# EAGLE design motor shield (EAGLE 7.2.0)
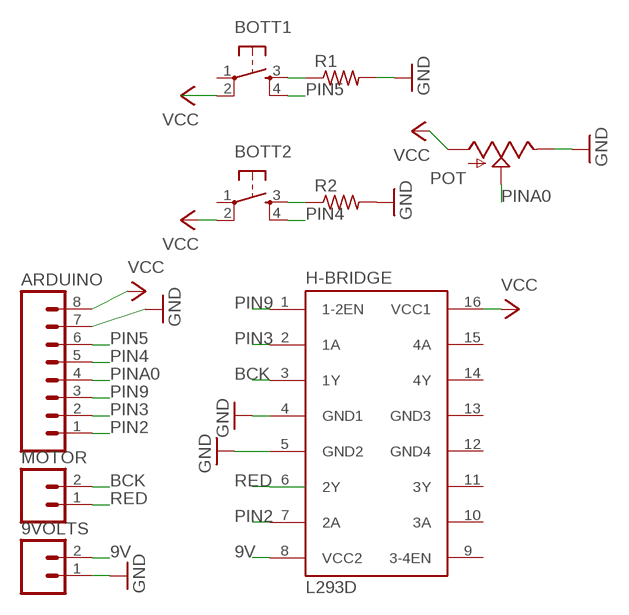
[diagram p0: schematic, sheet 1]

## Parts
9VOLTS  M02LOCK_LONGPADS  [1X02_LOCK_LONGPADS]
ARDUINO  M08LONGPADS  [1X08_LONGPADS]
BOTT1  6MM_SWITCH6MM_SWITCH  [6MM_SWITCH]
BOTT2  6MM_SWITCH6MM_SWITCH  [6MM_SWITCH]
H-BRIDGE  L293D  [DIL16]
MOTOR  M02LOCK_LONGPADS  [1X02_LOCK_LONGPADS]
POT  POT  [ALPS_POT]
R1  RESISTOR1206  [1206]
R2  RESISTOR1206  [1206]

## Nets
9V: 9VOLTS.2 H-BRIDGE.8(VCC2)
BCK: H-BRIDGE.3(1Y) MOTOR.2
GND: 9VOLTS.1 ARDUINO.7 H-BRIDGE.4(GND1) H-BRIDGE.5(GND2) POT.P$1(E) R1.2 R2.2
N$1: BOTT1.3(S) R1.1
N$2: BOTT2.3(S) R2.1
PIN2: ARDUINO.1 H-BRIDGE.7(2A)
PIN3: ARDUINO.2 H-BRIDGE.2(1A)
PIN4: ARDUINO.5 BOTT2.4(S1)
PIN5: ARDUINO.6 BOTT1.4(S1)
PIN9: ARDUINO.3 H-BRIDGE.1(1-2EN)
PINA0: ARDUINO.4 POT.P$2(S)
RED: H-BRIDGE.6(2Y) MOTOR.1
VCC: ARDUINO.8 BOTT1.2(P1) BOTT2.2(P1) H-BRIDGE.16(VCC1) POT.P$3(A)
Unconnected: BOTT1.1(P) BOTT2.1(P) H-BRIDGE.9(3-4EN) H-BRIDGE.10(3A) H-BRIDGE.11(3Y) H-BRIDGE.14(4Y) H-BRIDGE.15(4A)

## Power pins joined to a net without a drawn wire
GND3: H-BRIDGE.13(GND3)
GND4: H-BRIDGE.12(GND4)

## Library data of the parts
9VOLTS MOTOR = 01_SparkFun:M02: Header 2
ARDUINO = 01_SparkFun:M08: Header 8 Standard 8-pin 0.1" header. Use with straight break away headers (SKU : PRT-00116), right angle break away headers (PRT-00553), swiss pins (PRT-00743), machine pins (PRT-00117), and female headers (PRT-00115).
BOTT1 BOTT2 = 01_FAB_Hello:6MM_SWITCH: OMRON SWITCH
H-BRIDGE = st-microelectronics:L293D: PUSH-PULL 4 CHANNEL DRIVER; MPN: L293D; OC_FARNELL: 9589619; OC_NEWARK: 56P8249
POT = 01_SparkFun:POT
R1 R2 = 01_FAB_Hello:RESISTOR

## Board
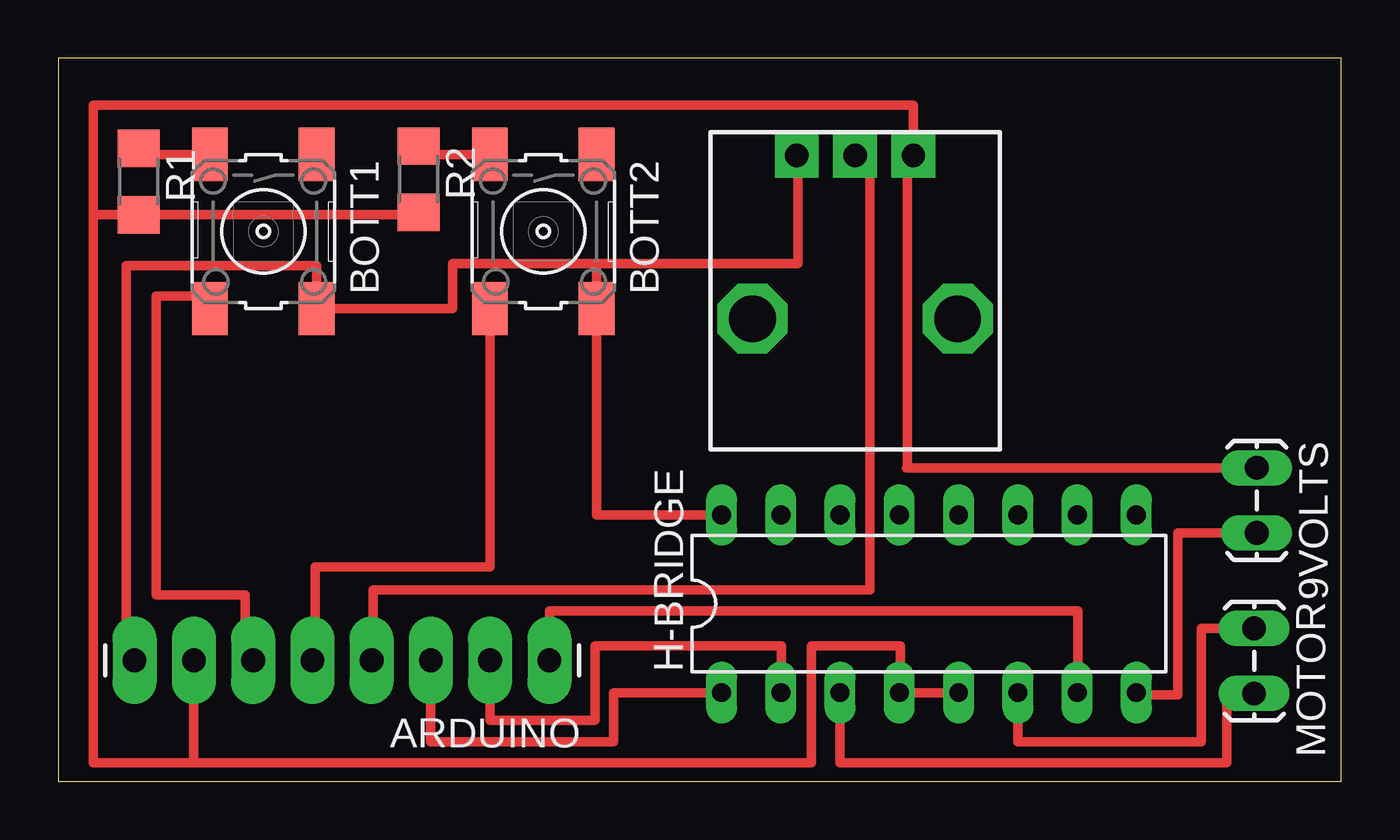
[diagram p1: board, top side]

Size 55 x 31 mm. Coordinates in mm from the lower left corner, seen from the top.
Outline: 0,0 55,0 55,31 0,31 0,0
Copper layers (1*16): Top 0.035mm / dielectric 1.5mm / Bottom 0.035mm
Design rules "default *": minimum track width 0.3mm, minimum drill 24mil, track to track 0.4mm, track to pad 0.4mm, pad to pad 0.4mm, via to via 0.4mm, smd to smd 0.4mm, copper to edge 40mil, drill to drill 8mil, minimum pad ring 10mil, minimum via ring 8mil, stop-mask expansion 4mil, vias tented up to drill 0mil, thermal gap 10mil

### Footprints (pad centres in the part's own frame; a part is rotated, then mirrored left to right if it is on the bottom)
1X02_LOCK_LONGPADS = drill 1.016 long: 1 -0.127,0; 2 2.667,0
1X08_LONGPADS = drill 1.016 pad 1.88 long: 1 0,0; 2 2.54,0; 3 5.08,0; 4 7.62,0; 5 10.16,0; 6 12.7,0; 7 15.24,0; 8 17.78,0
6MM_SWITCH = smd 2.286 x 1.524: 1 -3.302,2.286; 2 3.302,2.286; 3 -3.302,-2.286; 4 3.302,-2.286
DIL16 = drill 0.813 long: 1 -8.89,-3.81; 2 -6.35,-3.81; 3 -3.81,-3.81; 4 -1.27,-3.81; 5 1.27,-3.81; 6 3.81,-3.81; 7 6.35,-3.81; 8 8.89,-3.81; 9 8.89,3.81; 10 6.35,3.81; 11 3.81,3.81; 12 1.27,3.81; 13 -1.27,3.81; 14 -3.81,3.81; 15 -6.35,3.81; 16 -8.89,3.81
ALPS_POT = drill 1 pad 1.88 square: P$1 7,-2.5; P$2 7,0; P$3 7,2.5 | drill 2 octagon: P$4 0,-4.4; P$5 0,4.4
1206 = smd 1.6 x 1.803: 1 -1.422,0; 2 1.422,0

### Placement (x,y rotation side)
9VOLTS  51.38,13.31 270 top
ARDUINO  21.05,5.18 180 top
BOTT1  8.79,23.57 270 top
BOTT2  20.79,23.57 270 top
H-BRIDGE  37.33,7.61 0 top
MOTOR  51.27,6.43 270 top
POT  34.16,19.83 90 top
R1  3.45,25.71 270 top
R2  15.45,25.81 270 top

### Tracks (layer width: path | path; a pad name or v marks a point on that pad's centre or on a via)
9V
  Top 0.406: 9VOLTS.2 48,10.64 48,3.7 46.22,3.7 H-BRIDGE.8
BCK
  Top 0.406: MOTOR.2 50.1,3.76 50.1,0.8 33.52,0.8 H-BRIDGE.3
GND
  Top 0.406: 36.1,3.8 H-BRIDGE.4 | H-BRIDGE.5 36.1,3.8 | 36.1,3.8 36.1,5.8 32.3,5.8 32.3,0.8 5.81,0.8 | R2.2 15.45,24.29 R1.2 1.5,24.29 | 1.5,24.29 1.5,0.8 5.81,0.8 | 5.81,0.8 ARDUINO.7 | 36.36,13.44 36.4,13.44 | 36.4,13.44 9VOLTS.1 | 1.5,24.29 1.5,29 36.66,29 POT.P$1 36.4,26.83 36.4,13.44
N$1
  Top 0.406: BOTT1.3 3.45,26.87 R1.1
N$2
  Top 0.406: BOTT2.3 15.45,26.87 R2.1
PIN2
  Top 0.406: H-BRIDGE.7 43.7,3.8 43.7,7.3 21.05,7.3 ARDUINO.1
PIN3
  Top 0.406: H-BRIDGE.2 31,3.8 31,5.8 23,5.8 23,2.6 18.51,2.6 ARDUINO.2
PIN4
  Top 0.406: ARDUINO.5 11,5.18 11,9.2 18.5,9.2 BOTT2.4
PIN5
  Top 0.406: ARDUINO.6 8,5.18 8,8 4.2,8 4.2,20.8 6.5,20.8 BOTT1.4
PIN9
  Top 0.406: H-BRIDGE.1 23.8,3.8 23.8,1.7 15.97,1.7 ARDUINO.3
PINA0
  Top 0.406: ARDUINO.4 13.5,5.18 13.5,8.2 34.8,8.2 34.8,26.5 34.16,26.5 POT.P$2
RED
  Top 0.406: MOTOR.1 49,6.56 49,1.7 41.14,1.7 H-BRIDGE.6
VCC
  Top 0.406: 23.08,22.2 16.9,22.2 16.9,20.27 BOTT1.2 11.08,22.1 2.9,22.1 2.9,5.18 ARDUINO.8 | BOTT2.2 22.8,20.27 22.8,20.3 | H-BRIDGE.16 23.08,11.42 BOTT2.2 | POT.P$3 31.7,26.83 31.7,22.2 23.08,22.2 | 23.08,22.2 BOTT2.2

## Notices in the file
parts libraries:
01_SparkFun: Licensing: CC v3.0 Share-Alike You are welcome to use this library for commercial purposes.
